(* Logix 5000 AddOnInstructionDefinition export EipIoDataMapping_PAL_EIP; software revision 37.00 *)

TYPE PneumaticAutomationLink_UDT :
STRUCT
   sts_DiagnosticData : SINT;
   sts_DigitalInput_8pt_Module : SINT[16];
   sts_AnalogInput : INT[16];   // Raw Data
   sts_DigitalInput_16pt_Module : INT[8];
   sts_TemperatureInput : INT[16];   // Implied Decimal
   cmd_Valves : BOOL[128];   // Solenoids
   cmd_DigitalOutput_8pt_Module : SINT[16];
   cmd_DigitalOutput_6pt_Module : SINT[22];   // w/ Auxiliary Power
   cmd_AnalogOutput : INT[16];   // Raw Data
   cmd_DigitalOutput_16pt_Module : INT[8];
END_STRUCT
END_TYPE

ADD_ON_INSTRUCTION EipIoDataMapping_PAL_EIP   (* revision 1.0, vendor Automationdirect.com *)
// This Add-On Instruction unpacks raw Input Data (T->O) from an array and maps this data into meaningful device related status tags for the user. Likewise, the AOI also maps meaningful device related command tags and packs the data into the raw Output Data (O->T) array.
// The purpose of the Add-On Instruction is to simplify the mapping (packing/unpacking) of the raw Input/Output Data. For operation of the drive, the user must provide their own logic.
// Revision note:
// Created in v37.00.00
// Version: 1.0
// - Initial version of the new Add-On Instruction format.
// 2025/06/20
VAR_IN_OUT
   mod_EipInputData : _054B:PAL_EIP_D8303EE7:I:0; {required}   // Module defined using SINT data type
   mod_EipOutputData : _054B:PAL_EIP_3E1CE89C:O:0; {required}   // Module defined using SINT data type
   ref_InstanceOfPal : PneumaticAutomationLink_UDT; {required}   // Reference to an instance of the PneumaticAutomationLink_UDT
END_VAR

ROUTINE Logic   (* ladder *)
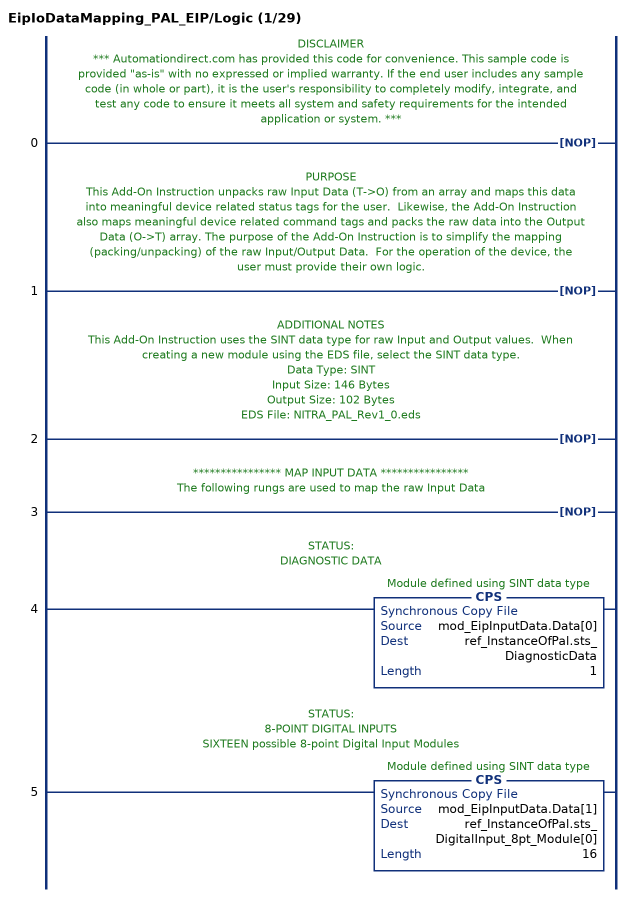
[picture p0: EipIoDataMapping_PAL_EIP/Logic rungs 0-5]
   // DISCLAIMER
   // *** Automationdirect.com has provided this code for convenience. This sample code is provided "as-is" with no expressed or implied warranty. If the end user includes any sample code (in whole or part), it is the user's responsibility to completely modify, integrate, and test any code to ensure it meets all system and safety requirements for the intended application or system. ***
   0: NOP();
   // PURPOSE
   // This Add-On Instruction unpacks raw Input Data (T->O) from an array and maps this data into meaningful device related status tags for the user.  Likewise, the Add-On Instruction also maps meaningful device related command tags and packs the raw data into the Output Data (O->T) array. The purpose of the Add-On Instruction is to simplify the mapping (packing/unpacking) of the raw Input/Output Data.  For the operation of the device, the user must provide their own logic.
   1: NOP();
   // ADDITIONAL NOTES
   // This Add-On Instruction uses the SINT data type for raw Input and Output values.  When creating a new module using the EDS file, select the SINT data type.
   // Data Type: SINT
   // Input Size: 146 Bytes
   // Output Size: 102 Bytes
   // EDS File: NITRA_PAL_Rev1_0.eds
   2: NOP();
   // **************** MAP INPUT DATA ****************
   // The following rungs are used to map the raw Input Data
   3: NOP();
   // STATUS:
   // DIAGNOSTIC DATA
   4: CPS(mod_EipInputData.Data[0],ref_InstanceOfPal.sts_DiagnosticData,1);
   // STATUS:
   // 8-POINT DIGITAL INPUTS
   // SIXTEEN possible 8-point Digital Input Modules
   5: CPS(mod_EipInputData.Data[1],ref_InstanceOfPal.sts_DigitalInput_8pt_Module[0],16);
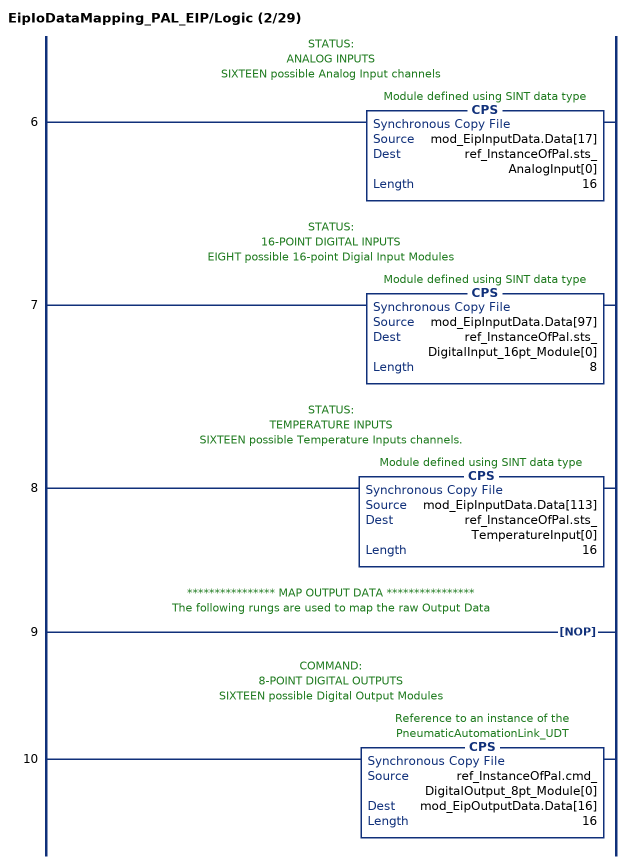
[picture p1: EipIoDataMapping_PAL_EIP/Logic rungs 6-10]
   // STATUS:
   // ANALOG INPUTS
   // SIXTEEN possible Analog Input channels
   6: CPS(mod_EipInputData.Data[17],ref_InstanceOfPal.sts_AnalogInput[0],16);
   // STATUS:
   // 16-POINT DIGITAL INPUTS
   // EIGHT possible 16-point Digial Input Modules
   7: CPS(mod_EipInputData.Data[97],ref_InstanceOfPal.sts_DigitalInput_16pt_Module[0],8);
   // STATUS:
   // TEMPERATURE INPUTS
   // SIXTEEN possible Temperature Inputs channels.
   8: CPS(mod_EipInputData.Data[113],ref_InstanceOfPal.sts_TemperatureInput[0],16);
   // **************** MAP OUTPUT DATA ****************
   // The following rungs are used to map the raw Output Data
   9: NOP();
   // COMMAND:
   // 8-POINT DIGITAL OUTPUTS
   // SIXTEEN possible Digital Output Modules
   10: CPS(ref_InstanceOfPal.cmd_DigitalOutput_8pt_Module[0],mod_EipOutputData.Data[16],16);
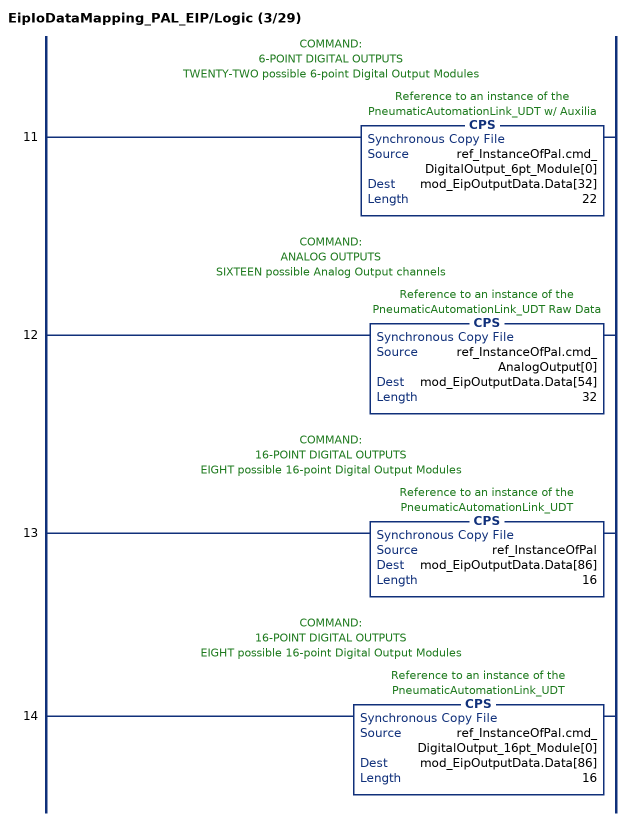
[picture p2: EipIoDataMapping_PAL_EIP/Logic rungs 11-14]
   // COMMAND:
   // 6-POINT DIGITAL OUTPUTS
   // TWENTY-TWO possible 6-point Digital Output Modules
   11: CPS(ref_InstanceOfPal.cmd_DigitalOutput_6pt_Module[0],mod_EipOutputData.Data[32],22);
   // COMMAND:
   // ANALOG OUTPUTS
   // SIXTEEN possible Analog Output channels
   12: CPS(ref_InstanceOfPal.cmd_AnalogOutput[0],mod_EipOutputData.Data[54],32);
   // COMMAND:
   // 16-POINT DIGITAL OUTPUTS
   // EIGHT possible 16-point Digital Output Modules
   13: CPS(ref_InstanceOfPal,mod_EipOutputData.Data[86],16);
   // COMMAND:
   // 16-POINT DIGITAL OUTPUTS
   // EIGHT possible 16-point Digital Output Modules
   14: CPS(ref_InstanceOfPal.cmd_DigitalOutput_16pt_Module[0],mod_EipOutputData.Data[86],16);
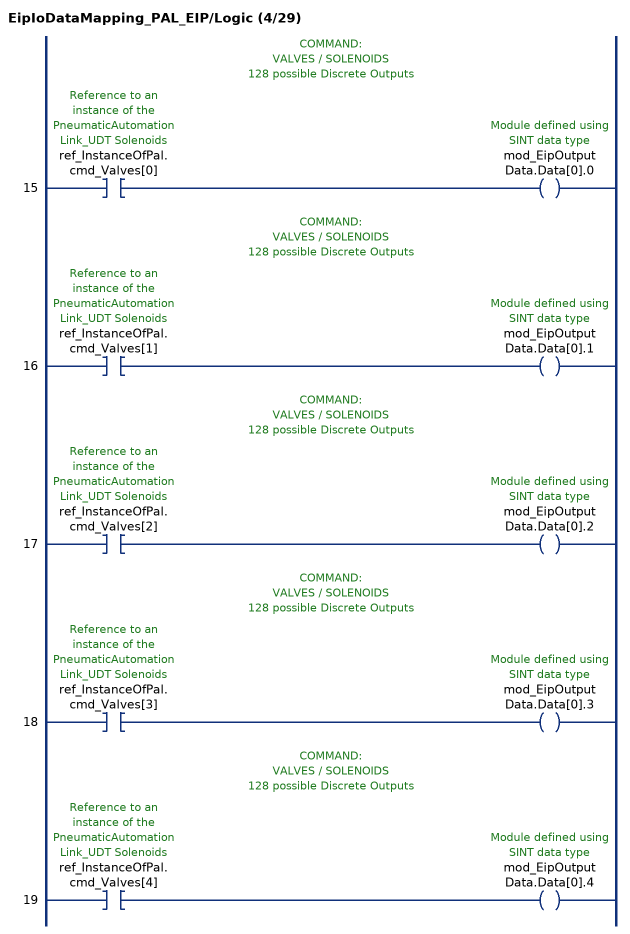
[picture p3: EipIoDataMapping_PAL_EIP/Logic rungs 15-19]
   // COMMAND:
   // VALVES / SOLENOIDS
   // 128 possible Discrete Outputs
   15: XIC(ref_InstanceOfPal.cmd_Valves[0])OTE(mod_EipOutputData.Data[0].0);
   // COMMAND:
   // VALVES / SOLENOIDS
   // 128 possible Discrete Outputs
   16: XIC(ref_InstanceOfPal.cmd_Valves[1])OTE(mod_EipOutputData.Data[0].1);
   // COMMAND:
   // VALVES / SOLENOIDS
   // 128 possible Discrete Outputs
   17: XIC(ref_InstanceOfPal.cmd_Valves[2])OTE(mod_EipOutputData.Data[0].2);
   // COMMAND:
   // VALVES / SOLENOIDS
   // 128 possible Discrete Outputs
   18: XIC(ref_InstanceOfPal.cmd_Valves[3])OTE(mod_EipOutputData.Data[0].3);
   // COMMAND:
   // VALVES / SOLENOIDS
   // 128 possible Discrete Outputs
   19: XIC(ref_InstanceOfPal.cmd_Valves[4])OTE(mod_EipOutputData.Data[0].4);
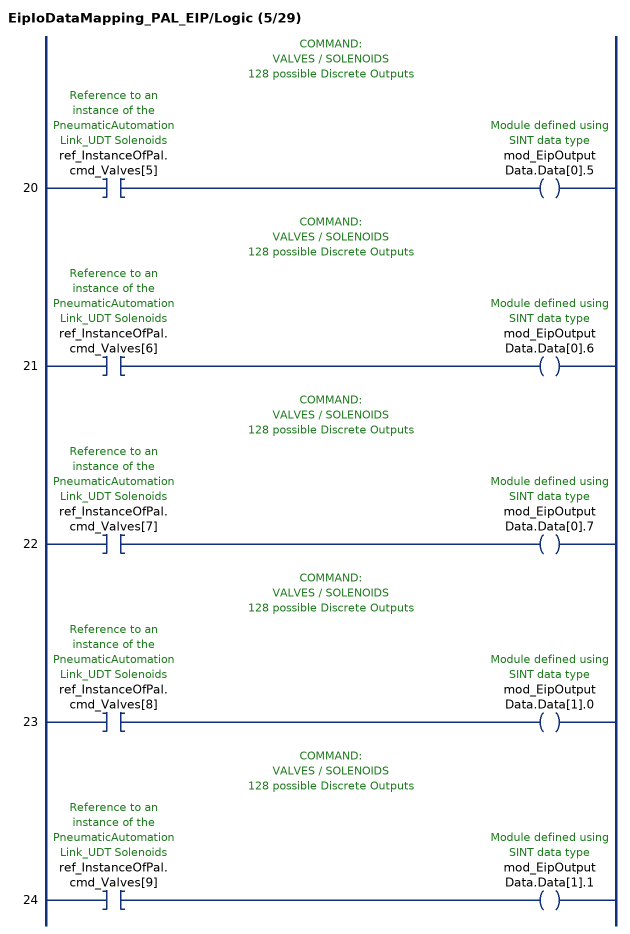
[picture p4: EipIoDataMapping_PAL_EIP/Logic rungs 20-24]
   // COMMAND:
   // VALVES / SOLENOIDS
   // 128 possible Discrete Outputs
   20: XIC(ref_InstanceOfPal.cmd_Valves[5])OTE(mod_EipOutputData.Data[0].5);
   // COMMAND:
   // VALVES / SOLENOIDS
   // 128 possible Discrete Outputs
   21: XIC(ref_InstanceOfPal.cmd_Valves[6])OTE(mod_EipOutputData.Data[0].6);
   // COMMAND:
   // VALVES / SOLENOIDS
   // 128 possible Discrete Outputs
   22: XIC(ref_InstanceOfPal.cmd_Valves[7])OTE(mod_EipOutputData.Data[0].7);
   // COMMAND:
   // VALVES / SOLENOIDS
   // 128 possible Discrete Outputs
   23: XIC(ref_InstanceOfPal.cmd_Valves[8])OTE(mod_EipOutputData.Data[1].0);
   // COMMAND:
   // VALVES / SOLENOIDS
   // 128 possible Discrete Outputs
   24: XIC(ref_InstanceOfPal.cmd_Valves[9])OTE(mod_EipOutputData.Data[1].1);
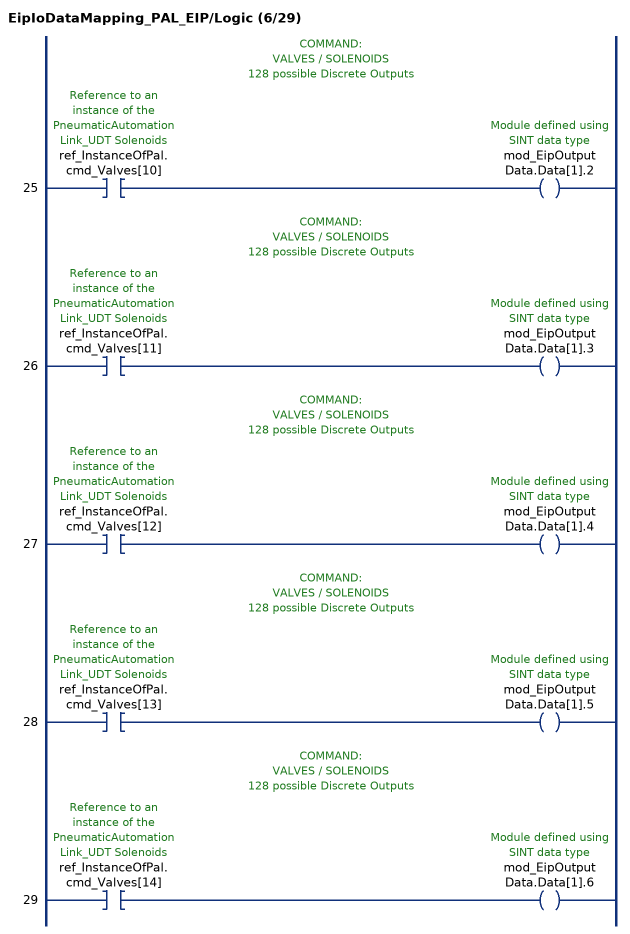
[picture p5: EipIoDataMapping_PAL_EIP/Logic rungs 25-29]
   // COMMAND:
   // VALVES / SOLENOIDS
   // 128 possible Discrete Outputs
   25: XIC(ref_InstanceOfPal.cmd_Valves[10])OTE(mod_EipOutputData.Data[1].2);
   // COMMAND:
   // VALVES / SOLENOIDS
   // 128 possible Discrete Outputs
   26: XIC(ref_InstanceOfPal.cmd_Valves[11])OTE(mod_EipOutputData.Data[1].3);
   // COMMAND:
   // VALVES / SOLENOIDS
   // 128 possible Discrete Outputs
   27: XIC(ref_InstanceOfPal.cmd_Valves[12])OTE(mod_EipOutputData.Data[1].4);
   // COMMAND:
   // VALVES / SOLENOIDS
   // 128 possible Discrete Outputs
   28: XIC(ref_InstanceOfPal.cmd_Valves[13])OTE(mod_EipOutputData.Data[1].5);
   // COMMAND:
   // VALVES / SOLENOIDS
   // 128 possible Discrete Outputs
   29: XIC(ref_InstanceOfPal.cmd_Valves[14])OTE(mod_EipOutputData.Data[1].6);
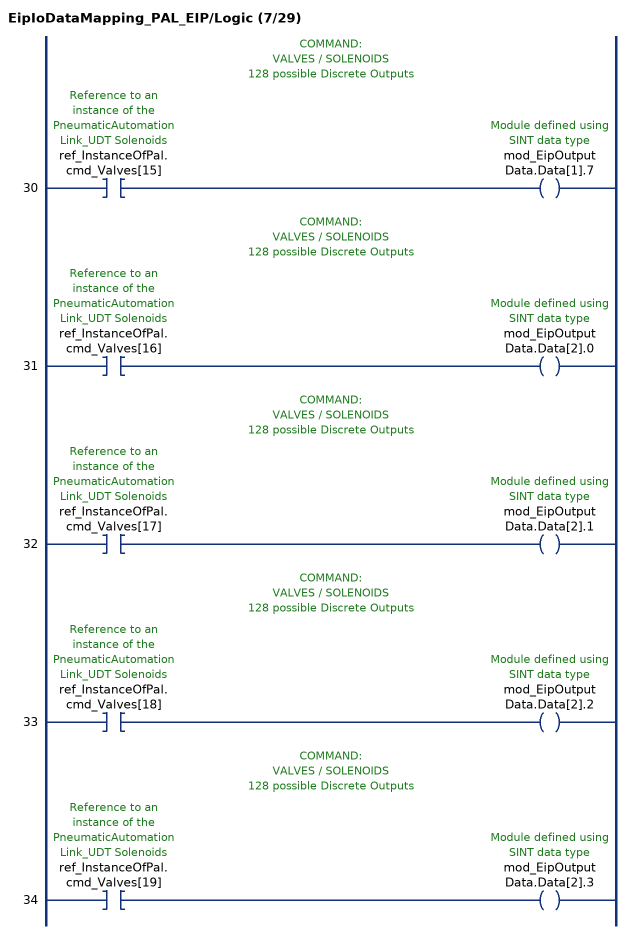
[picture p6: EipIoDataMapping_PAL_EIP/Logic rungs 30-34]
   // COMMAND:
   // VALVES / SOLENOIDS
   // 128 possible Discrete Outputs
   30: XIC(ref_InstanceOfPal.cmd_Valves[15])OTE(mod_EipOutputData.Data[1].7);
   // COMMAND:
   // VALVES / SOLENOIDS
   // 128 possible Discrete Outputs
   31: XIC(ref_InstanceOfPal.cmd_Valves[16])OTE(mod_EipOutputData.Data[2].0);
   // COMMAND:
   // VALVES / SOLENOIDS
   // 128 possible Discrete Outputs
   32: XIC(ref_InstanceOfPal.cmd_Valves[17])OTE(mod_EipOutputData.Data[2].1);
   // COMMAND:
   // VALVES / SOLENOIDS
   // 128 possible Discrete Outputs
   33: XIC(ref_InstanceOfPal.cmd_Valves[18])OTE(mod_EipOutputData.Data[2].2);
   // COMMAND:
   // VALVES / SOLENOIDS
   // 128 possible Discrete Outputs
   34: XIC(ref_InstanceOfPal.cmd_Valves[19])OTE(mod_EipOutputData.Data[2].3);
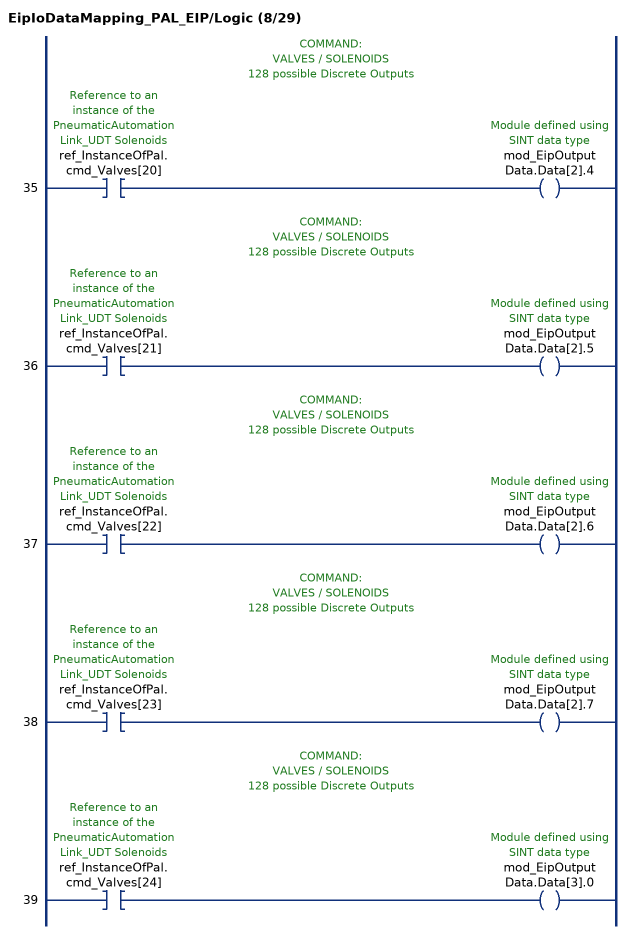
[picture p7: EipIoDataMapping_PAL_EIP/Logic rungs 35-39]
   // COMMAND:
   // VALVES / SOLENOIDS
   // 128 possible Discrete Outputs
   35: XIC(ref_InstanceOfPal.cmd_Valves[20])OTE(mod_EipOutputData.Data[2].4);
   // COMMAND:
   // VALVES / SOLENOIDS
   // 128 possible Discrete Outputs
   36: XIC(ref_InstanceOfPal.cmd_Valves[21])OTE(mod_EipOutputData.Data[2].5);
   // COMMAND:
   // VALVES / SOLENOIDS
   // 128 possible Discrete Outputs
   37: XIC(ref_InstanceOfPal.cmd_Valves[22])OTE(mod_EipOutputData.Data[2].6);
   // COMMAND:
   // VALVES / SOLENOIDS
   // 128 possible Discrete Outputs
   38: XIC(ref_InstanceOfPal.cmd_Valves[23])OTE(mod_EipOutputData.Data[2].7);
   // COMMAND:
   // VALVES / SOLENOIDS
   // 128 possible Discrete Outputs
   39: XIC(ref_InstanceOfPal.cmd_Valves[24])OTE(mod_EipOutputData.Data[3].0);
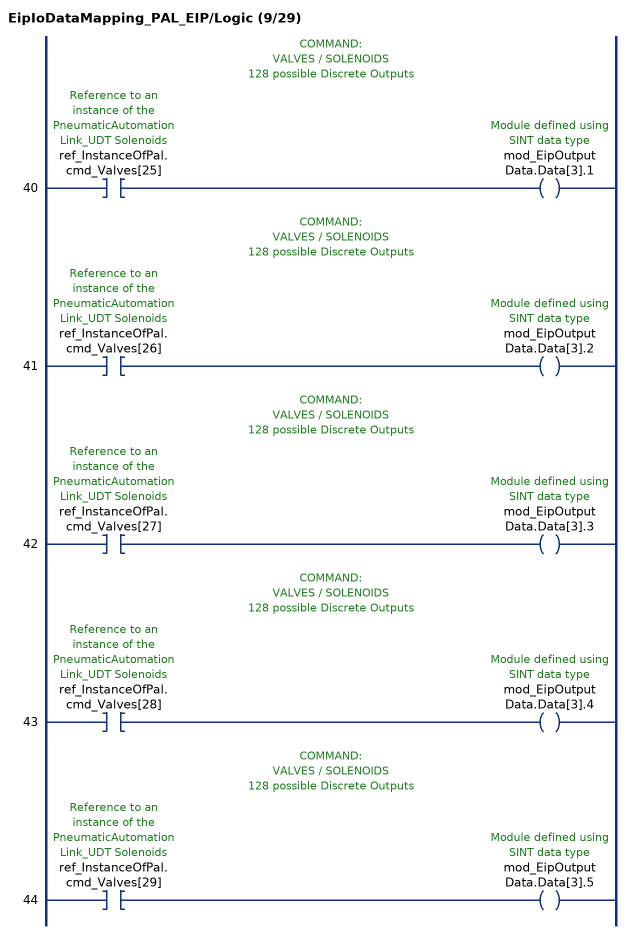
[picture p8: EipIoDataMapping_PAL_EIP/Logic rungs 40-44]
   // COMMAND:
   // VALVES / SOLENOIDS
   // 128 possible Discrete Outputs
   40: XIC(ref_InstanceOfPal.cmd_Valves[25])OTE(mod_EipOutputData.Data[3].1);
   // COMMAND:
   // VALVES / SOLENOIDS
   // 128 possible Discrete Outputs
   41: XIC(ref_InstanceOfPal.cmd_Valves[26])OTE(mod_EipOutputData.Data[3].2);
   // COMMAND:
   // VALVES / SOLENOIDS
   // 128 possible Discrete Outputs
   42: XIC(ref_InstanceOfPal.cmd_Valves[27])OTE(mod_EipOutputData.Data[3].3);
   // COMMAND:
   // VALVES / SOLENOIDS
   // 128 possible Discrete Outputs
   43: XIC(ref_InstanceOfPal.cmd_Valves[28])OTE(mod_EipOutputData.Data[3].4);
   // COMMAND:
   // VALVES / SOLENOIDS
   // 128 possible Discrete Outputs
   44: XIC(ref_InstanceOfPal.cmd_Valves[29])OTE(mod_EipOutputData.Data[3].5);
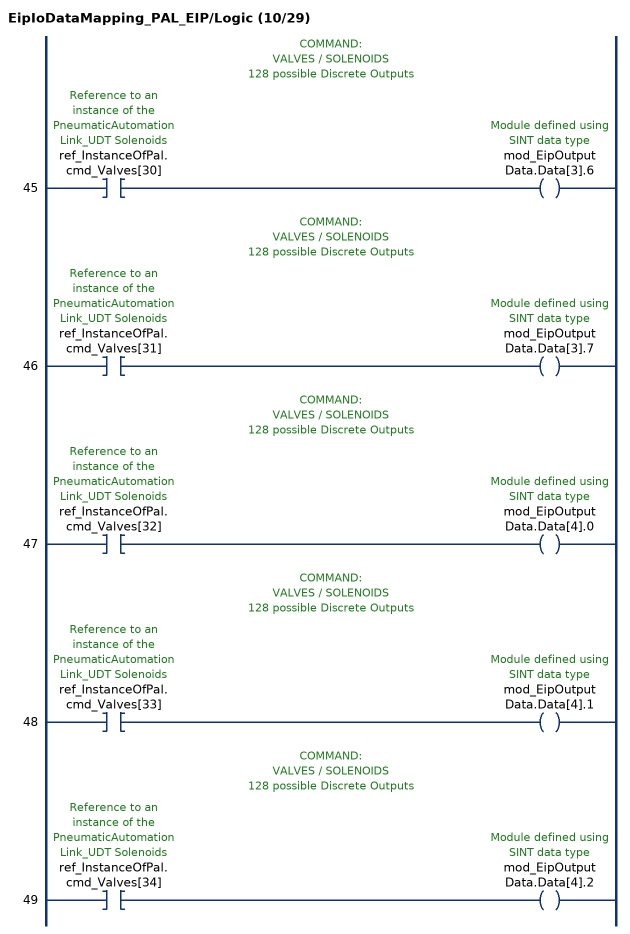
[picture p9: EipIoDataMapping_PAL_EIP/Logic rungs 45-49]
   // COMMAND:
   // VALVES / SOLENOIDS
   // 128 possible Discrete Outputs
   45: XIC(ref_InstanceOfPal.cmd_Valves[30])OTE(mod_EipOutputData.Data[3].6);
   // COMMAND:
   // VALVES / SOLENOIDS
   // 128 possible Discrete Outputs
   46: XIC(ref_InstanceOfPal.cmd_Valves[31])OTE(mod_EipOutputData.Data[3].7);
   // COMMAND:
   // VALVES / SOLENOIDS
   // 128 possible Discrete Outputs
   47: XIC(ref_InstanceOfPal.cmd_Valves[32])OTE(mod_EipOutputData.Data[4].0);
   // COMMAND:
   // VALVES / SOLENOIDS
   // 128 possible Discrete Outputs
   48: XIC(ref_InstanceOfPal.cmd_Valves[33])OTE(mod_EipOutputData.Data[4].1);
   // COMMAND:
   // VALVES / SOLENOIDS
   // 128 possible Discrete Outputs
   49: XIC(ref_InstanceOfPal.cmd_Valves[34])OTE(mod_EipOutputData.Data[4].2);
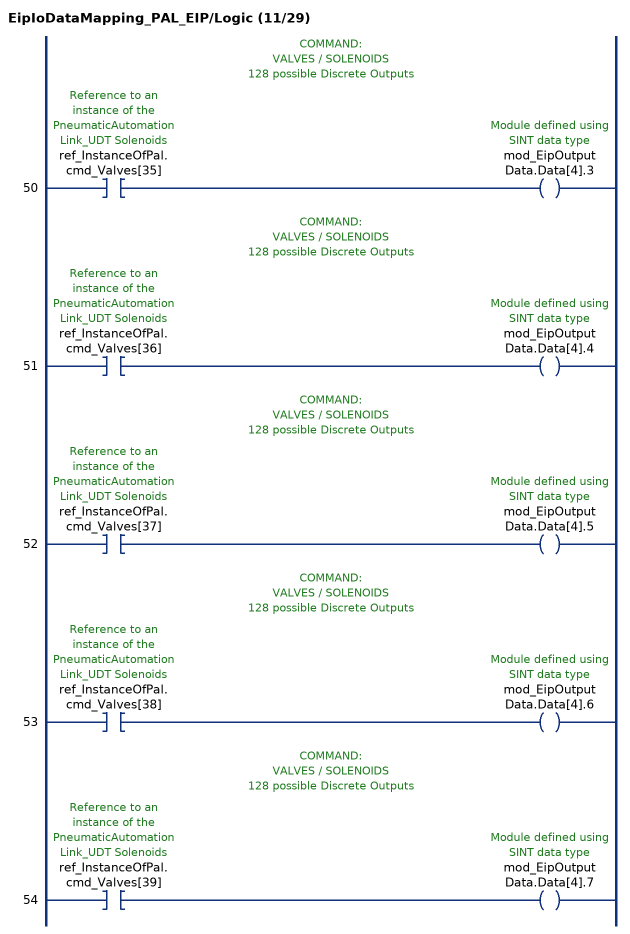
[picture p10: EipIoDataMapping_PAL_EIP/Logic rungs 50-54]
   // COMMAND:
   // VALVES / SOLENOIDS
   // 128 possible Discrete Outputs
   50: XIC(ref_InstanceOfPal.cmd_Valves[35])OTE(mod_EipOutputData.Data[4].3);
   // COMMAND:
   // VALVES / SOLENOIDS
   // 128 possible Discrete Outputs
   51: XIC(ref_InstanceOfPal.cmd_Valves[36])OTE(mod_EipOutputData.Data[4].4);
   // COMMAND:
   // VALVES / SOLENOIDS
   // 128 possible Discrete Outputs
   52: XIC(ref_InstanceOfPal.cmd_Valves[37])OTE(mod_EipOutputData.Data[4].5);
   // COMMAND:
   // VALVES / SOLENOIDS
   // 128 possible Discrete Outputs
   53: XIC(ref_InstanceOfPal.cmd_Valves[38])OTE(mod_EipOutputData.Data[4].6);
   // COMMAND:
   // VALVES / SOLENOIDS
   // 128 possible Discrete Outputs
   54: XIC(ref_InstanceOfPal.cmd_Valves[39])OTE(mod_EipOutputData.Data[4].7);
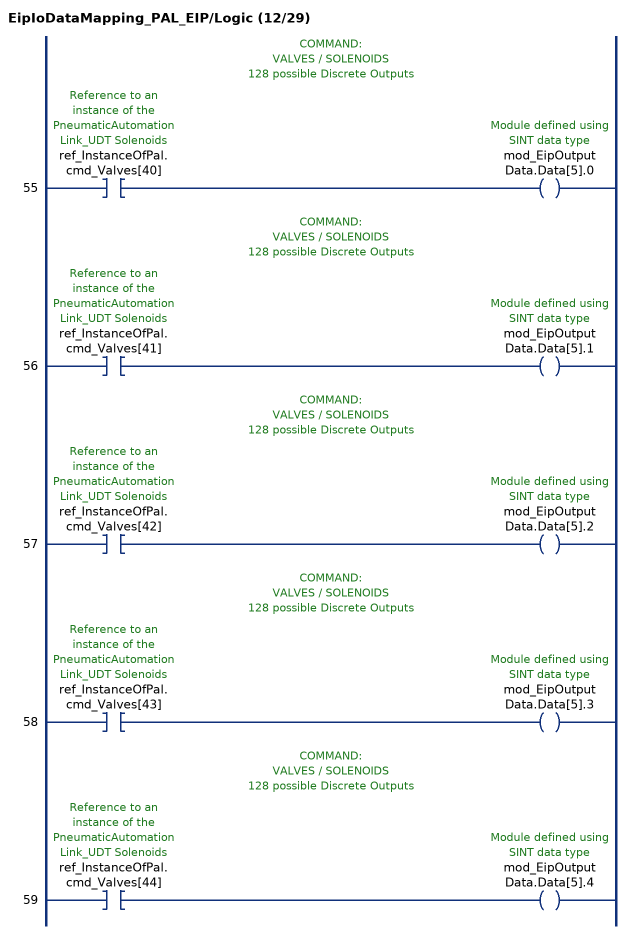
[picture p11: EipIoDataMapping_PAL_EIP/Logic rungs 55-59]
   // COMMAND:
   // VALVES / SOLENOIDS
   // 128 possible Discrete Outputs
   55: XIC(ref_InstanceOfPal.cmd_Valves[40])OTE(mod_EipOutputData.Data[5].0);
   // COMMAND:
   // VALVES / SOLENOIDS
   // 128 possible Discrete Outputs
   56: XIC(ref_InstanceOfPal.cmd_Valves[41])OTE(mod_EipOutputData.Data[5].1);
   // COMMAND:
   // VALVES / SOLENOIDS
   // 128 possible Discrete Outputs
   57: XIC(ref_InstanceOfPal.cmd_Valves[42])OTE(mod_EipOutputData.Data[5].2);
   // COMMAND:
   // VALVES / SOLENOIDS
   // 128 possible Discrete Outputs
   58: XIC(ref_InstanceOfPal.cmd_Valves[43])OTE(mod_EipOutputData.Data[5].3);
   // COMMAND:
   // VALVES / SOLENOIDS
   // 128 possible Discrete Outputs
   59: XIC(ref_InstanceOfPal.cmd_Valves[44])OTE(mod_EipOutputData.Data[5].4);
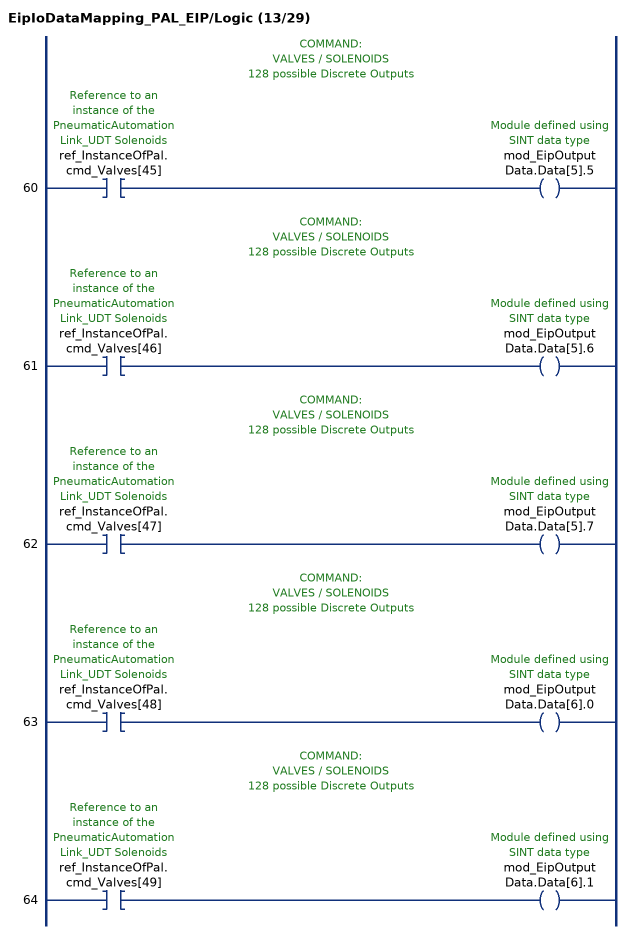
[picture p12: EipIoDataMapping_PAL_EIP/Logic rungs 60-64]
   // COMMAND:
   // VALVES / SOLENOIDS
   // 128 possible Discrete Outputs
   60: XIC(ref_InstanceOfPal.cmd_Valves[45])OTE(mod_EipOutputData.Data[5].5);
   // COMMAND:
   // VALVES / SOLENOIDS
   // 128 possible Discrete Outputs
   61: XIC(ref_InstanceOfPal.cmd_Valves[46])OTE(mod_EipOutputData.Data[5].6);
   // COMMAND:
   // VALVES / SOLENOIDS
   // 128 possible Discrete Outputs
   62: XIC(ref_InstanceOfPal.cmd_Valves[47])OTE(mod_EipOutputData.Data[5].7);
   // COMMAND:
   // VALVES / SOLENOIDS
   // 128 possible Discrete Outputs
   63: XIC(ref_InstanceOfPal.cmd_Valves[48])OTE(mod_EipOutputData.Data[6].0);
   // COMMAND:
   // VALVES / SOLENOIDS
   // 128 possible Discrete Outputs
   64: XIC(ref_InstanceOfPal.cmd_Valves[49])OTE(mod_EipOutputData.Data[6].1);
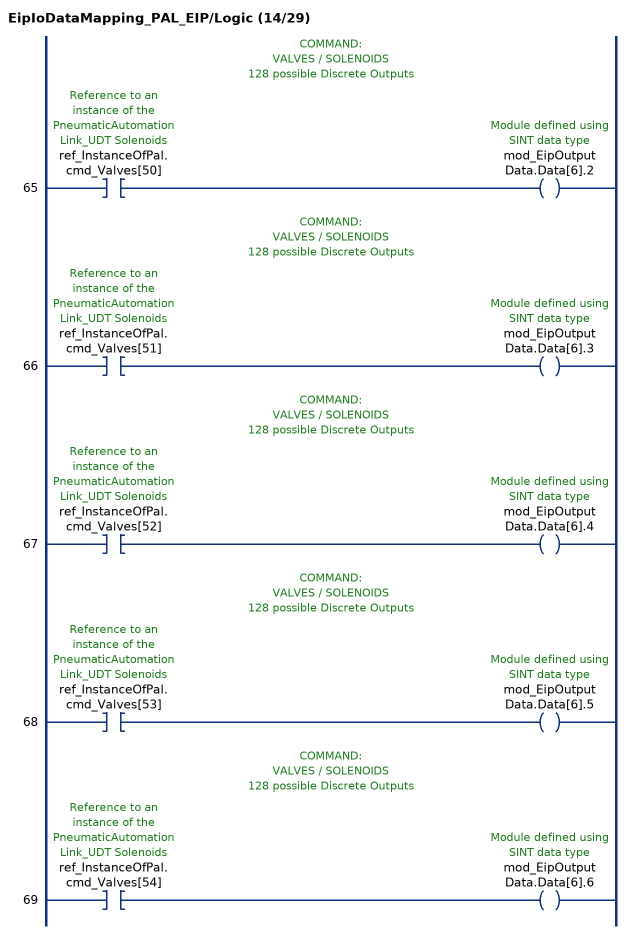
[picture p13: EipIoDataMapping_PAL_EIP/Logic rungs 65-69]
   // COMMAND:
   // VALVES / SOLENOIDS
   // 128 possible Discrete Outputs
   65: XIC(ref_InstanceOfPal.cmd_Valves[50])OTE(mod_EipOutputData.Data[6].2);
   // COMMAND:
   // VALVES / SOLENOIDS
   // 128 possible Discrete Outputs
   66: XIC(ref_InstanceOfPal.cmd_Valves[51])OTE(mod_EipOutputData.Data[6].3);
   // COMMAND:
   // VALVES / SOLENOIDS
   // 128 possible Discrete Outputs
   67: XIC(ref_InstanceOfPal.cmd_Valves[52])OTE(mod_EipOutputData.Data[6].4);
   // COMMAND:
   // VALVES / SOLENOIDS
   // 128 possible Discrete Outputs
   68: XIC(ref_InstanceOfPal.cmd_Valves[53])OTE(mod_EipOutputData.Data[6].5);
   // COMMAND:
   // VALVES / SOLENOIDS
   // 128 possible Discrete Outputs
   69: XIC(ref_InstanceOfPal.cmd_Valves[54])OTE(mod_EipOutputData.Data[6].6);
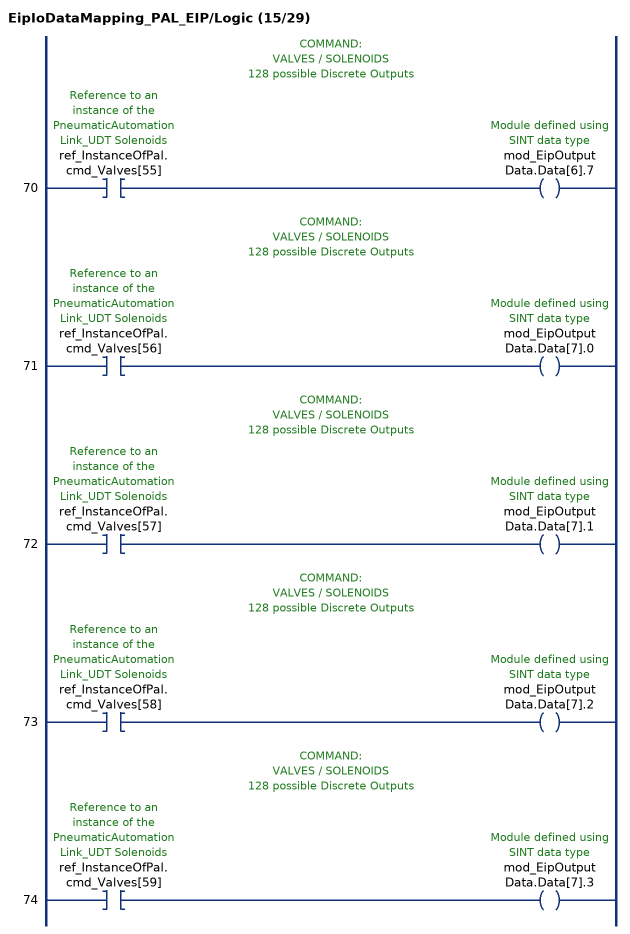
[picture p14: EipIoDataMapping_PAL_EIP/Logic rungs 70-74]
   // COMMAND:
   // VALVES / SOLENOIDS
   // 128 possible Discrete Outputs
   70: XIC(ref_InstanceOfPal.cmd_Valves[55])OTE(mod_EipOutputData.Data[6].7);
   // COMMAND:
   // VALVES / SOLENOIDS
   // 128 possible Discrete Outputs
   71: XIC(ref_InstanceOfPal.cmd_Valves[56])OTE(mod_EipOutputData.Data[7].0);
   // COMMAND:
   // VALVES / SOLENOIDS
   // 128 possible Discrete Outputs
   72: XIC(ref_InstanceOfPal.cmd_Valves[57])OTE(mod_EipOutputData.Data[7].1);
   // COMMAND:
   // VALVES / SOLENOIDS
   // 128 possible Discrete Outputs
   73: XIC(ref_InstanceOfPal.cmd_Valves[58])OTE(mod_EipOutputData.Data[7].2);
   // COMMAND:
   // VALVES / SOLENOIDS
   // 128 possible Discrete Outputs
   74: XIC(ref_InstanceOfPal.cmd_Valves[59])OTE(mod_EipOutputData.Data[7].3);
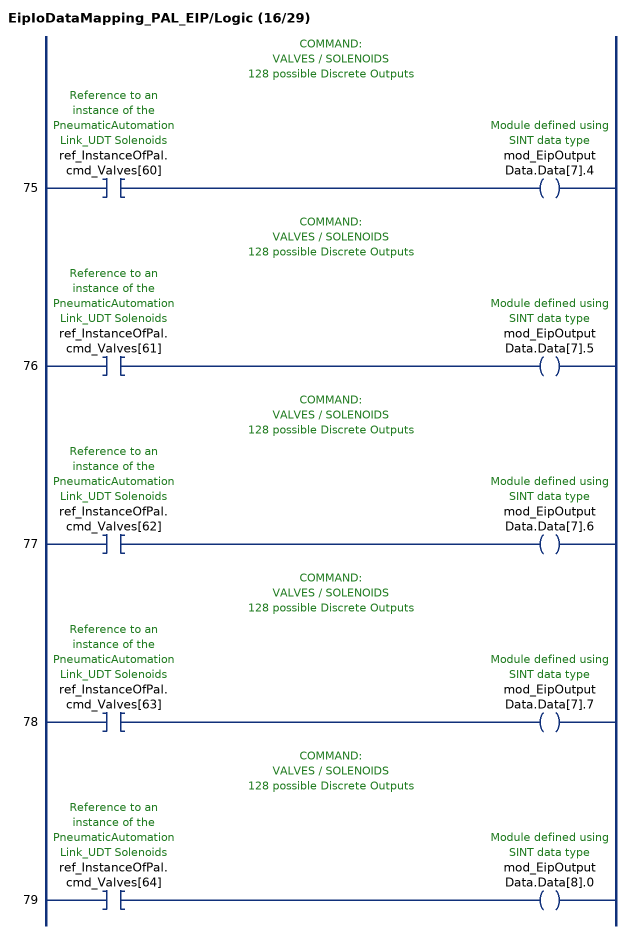
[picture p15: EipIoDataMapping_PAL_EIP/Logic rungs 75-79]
   // COMMAND:
   // VALVES / SOLENOIDS
   // 128 possible Discrete Outputs
   75: XIC(ref_InstanceOfPal.cmd_Valves[60])OTE(mod_EipOutputData.Data[7].4);
   // COMMAND:
   // VALVES / SOLENOIDS
   // 128 possible Discrete Outputs
   76: XIC(ref_InstanceOfPal.cmd_Valves[61])OTE(mod_EipOutputData.Data[7].5);
   // COMMAND:
   // VALVES / SOLENOIDS
   // 128 possible Discrete Outputs
   77: XIC(ref_InstanceOfPal.cmd_Valves[62])OTE(mod_EipOutputData.Data[7].6);
   // COMMAND:
   // VALVES / SOLENOIDS
   // 128 possible Discrete Outputs
   78: XIC(ref_InstanceOfPal.cmd_Valves[63])OTE(mod_EipOutputData.Data[7].7);
   // COMMAND:
   // VALVES / SOLENOIDS
   // 128 possible Discrete Outputs
   79: XIC(ref_InstanceOfPal.cmd_Valves[64])OTE(mod_EipOutputData.Data[8].0);
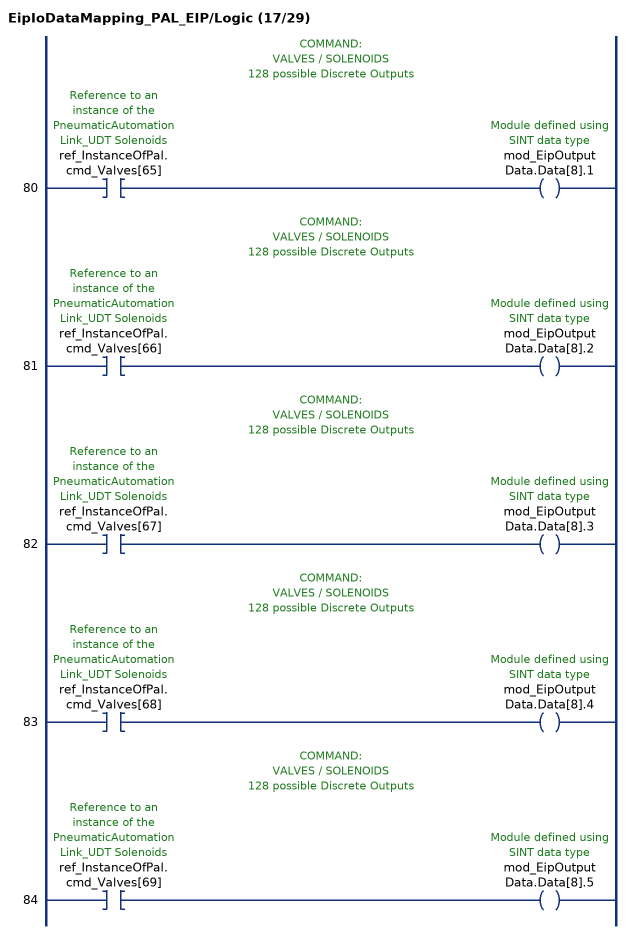
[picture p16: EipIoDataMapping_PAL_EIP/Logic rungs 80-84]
   // COMMAND:
   // VALVES / SOLENOIDS
   // 128 possible Discrete Outputs
   80: XIC(ref_InstanceOfPal.cmd_Valves[65])OTE(mod_EipOutputData.Data[8].1);
   // COMMAND:
   // VALVES / SOLENOIDS
   // 128 possible Discrete Outputs
   81: XIC(ref_InstanceOfPal.cmd_Valves[66])OTE(mod_EipOutputData.Data[8].2);
   // COMMAND:
   // VALVES / SOLENOIDS
   // 128 possible Discrete Outputs
   82: XIC(ref_InstanceOfPal.cmd_Valves[67])OTE(mod_EipOutputData.Data[8].3);
   // COMMAND:
   // VALVES / SOLENOIDS
   // 128 possible Discrete Outputs
   83: XIC(ref_InstanceOfPal.cmd_Valves[68])OTE(mod_EipOutputData.Data[8].4);
   // COMMAND:
   // VALVES / SOLENOIDS
   // 128 possible Discrete Outputs
   84: XIC(ref_InstanceOfPal.cmd_Valves[69])OTE(mod_EipOutputData.Data[8].5);
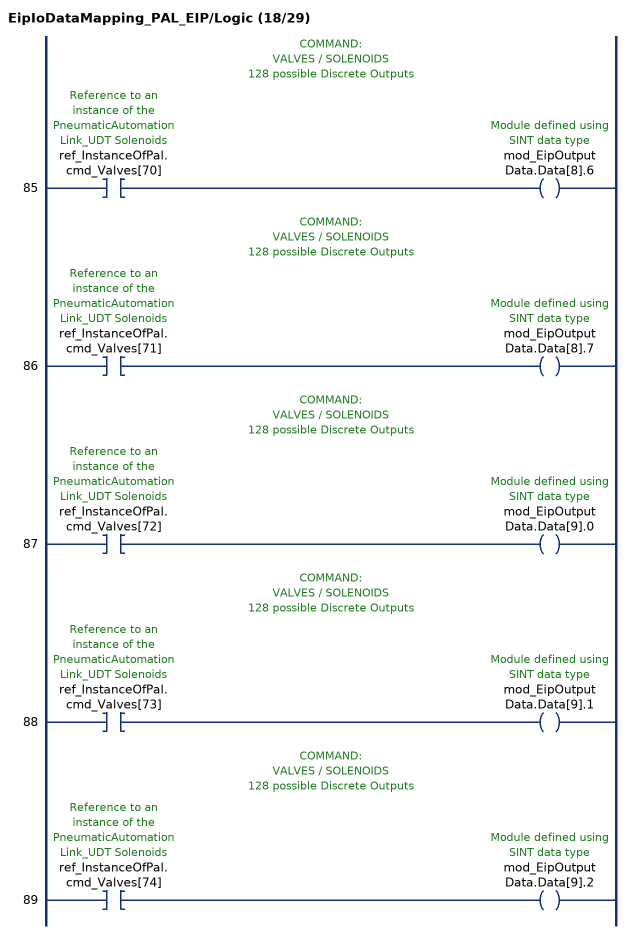
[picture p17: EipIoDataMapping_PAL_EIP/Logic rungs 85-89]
   // COMMAND:
   // VALVES / SOLENOIDS
   // 128 possible Discrete Outputs
   85: XIC(ref_InstanceOfPal.cmd_Valves[70])OTE(mod_EipOutputData.Data[8].6);
   // COMMAND:
   // VALVES / SOLENOIDS
   // 128 possible Discrete Outputs
   86: XIC(ref_InstanceOfPal.cmd_Valves[71])OTE(mod_EipOutputData.Data[8].7);
   // COMMAND:
   // VALVES / SOLENOIDS
   // 128 possible Discrete Outputs
   87: XIC(ref_InstanceOfPal.cmd_Valves[72])OTE(mod_EipOutputData.Data[9].0);
   // COMMAND:
   // VALVES / SOLENOIDS
   // 128 possible Discrete Outputs
   88: XIC(ref_InstanceOfPal.cmd_Valves[73])OTE(mod_EipOutputData.Data[9].1);
   // COMMAND:
   // VALVES / SOLENOIDS
   // 128 possible Discrete Outputs
   89: XIC(ref_InstanceOfPal.cmd_Valves[74])OTE(mod_EipOutputData.Data[9].2);
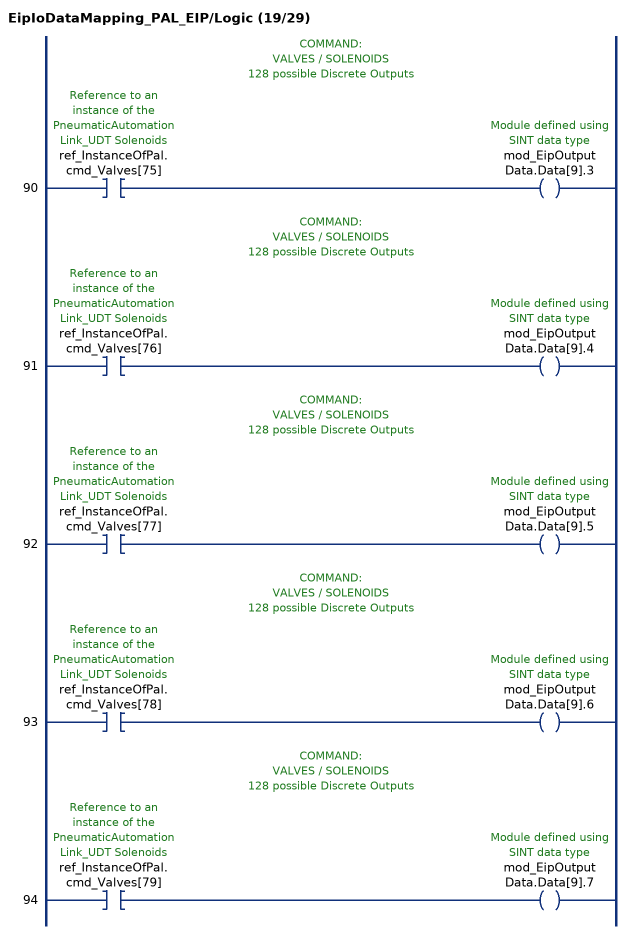
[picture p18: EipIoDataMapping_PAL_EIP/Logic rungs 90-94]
   // COMMAND:
   // VALVES / SOLENOIDS
   // 128 possible Discrete Outputs
   90: XIC(ref_InstanceOfPal.cmd_Valves[75])OTE(mod_EipOutputData.Data[9].3);
   // COMMAND:
   // VALVES / SOLENOIDS
   // 128 possible Discrete Outputs
   91: XIC(ref_InstanceOfPal.cmd_Valves[76])OTE(mod_EipOutputData.Data[9].4);
   // COMMAND:
   // VALVES / SOLENOIDS
   // 128 possible Discrete Outputs
   92: XIC(ref_InstanceOfPal.cmd_Valves[77])OTE(mod_EipOutputData.Data[9].5);
   // COMMAND:
   // VALVES / SOLENOIDS
   // 128 possible Discrete Outputs
   93: XIC(ref_InstanceOfPal.cmd_Valves[78])OTE(mod_EipOutputData.Data[9].6);
   // COMMAND:
   // VALVES / SOLENOIDS
   // 128 possible Discrete Outputs
   94: XIC(ref_InstanceOfPal.cmd_Valves[79])OTE(mod_EipOutputData.Data[9].7);
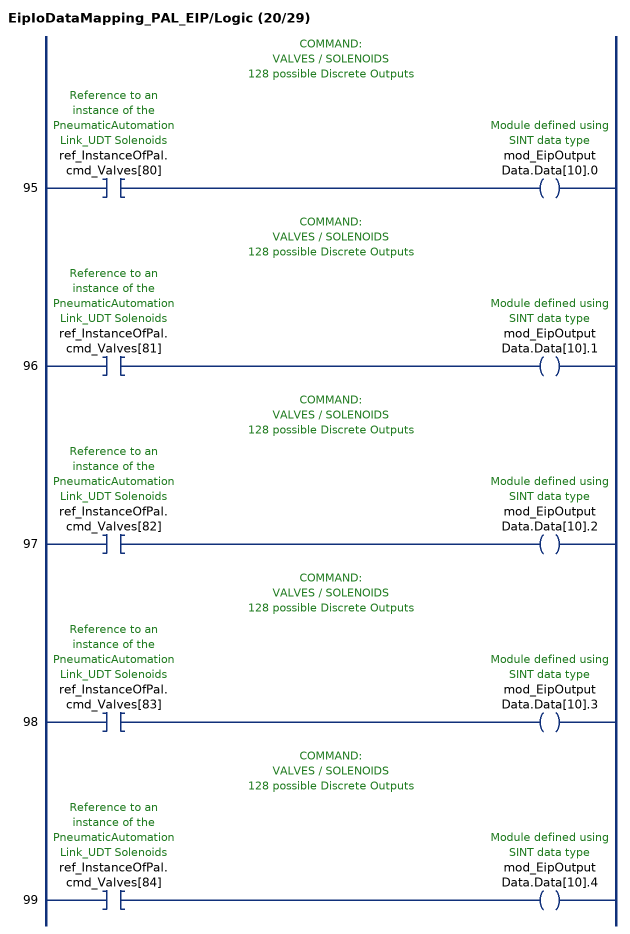
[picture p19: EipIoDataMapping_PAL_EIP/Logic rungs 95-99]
   // COMMAND:
   // VALVES / SOLENOIDS
   // 128 possible Discrete Outputs
   95: XIC(ref_InstanceOfPal.cmd_Valves[80])OTE(mod_EipOutputData.Data[10].0);
   // COMMAND:
   // VALVES / SOLENOIDS
   // 128 possible Discrete Outputs
   96: XIC(ref_InstanceOfPal.cmd_Valves[81])OTE(mod_EipOutputData.Data[10].1);
   // COMMAND:
   // VALVES / SOLENOIDS
   // 128 possible Discrete Outputs
   97: XIC(ref_InstanceOfPal.cmd_Valves[82])OTE(mod_EipOutputData.Data[10].2);
   // COMMAND:
   // VALVES / SOLENOIDS
   // 128 possible Discrete Outputs
   98: XIC(ref_InstanceOfPal.cmd_Valves[83])OTE(mod_EipOutputData.Data[10].3);
   // COMMAND:
   // VALVES / SOLENOIDS
   // 128 possible Discrete Outputs
   99: XIC(ref_InstanceOfPal.cmd_Valves[84])OTE(mod_EipOutputData.Data[10].4);
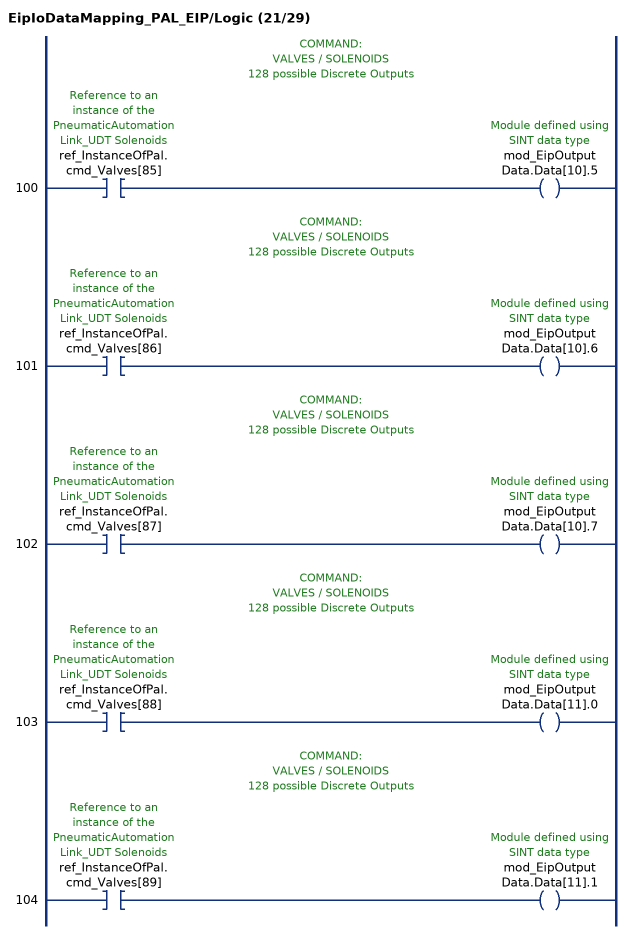
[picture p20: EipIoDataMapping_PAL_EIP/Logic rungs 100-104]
   // COMMAND:
   // VALVES / SOLENOIDS
   // 128 possible Discrete Outputs
   100: XIC(ref_InstanceOfPal.cmd_Valves[85])OTE(mod_EipOutputData.Data[10].5);
   // COMMAND:
   // VALVES / SOLENOIDS
   // 128 possible Discrete Outputs
   101: XIC(ref_InstanceOfPal.cmd_Valves[86])OTE(mod_EipOutputData.Data[10].6);
   // COMMAND:
   // VALVES / SOLENOIDS
   // 128 possible Discrete Outputs
   102: XIC(ref_InstanceOfPal.cmd_Valves[87])OTE(mod_EipOutputData.Data[10].7);
   // COMMAND:
   // VALVES / SOLENOIDS
   // 128 possible Discrete Outputs
   103: XIC(ref_InstanceOfPal.cmd_Valves[88])OTE(mod_EipOutputData.Data[11].0);
   // COMMAND:
   // VALVES / SOLENOIDS
   // 128 possible Discrete Outputs
   104: XIC(ref_InstanceOfPal.cmd_Valves[89])OTE(mod_EipOutputData.Data[11].1);
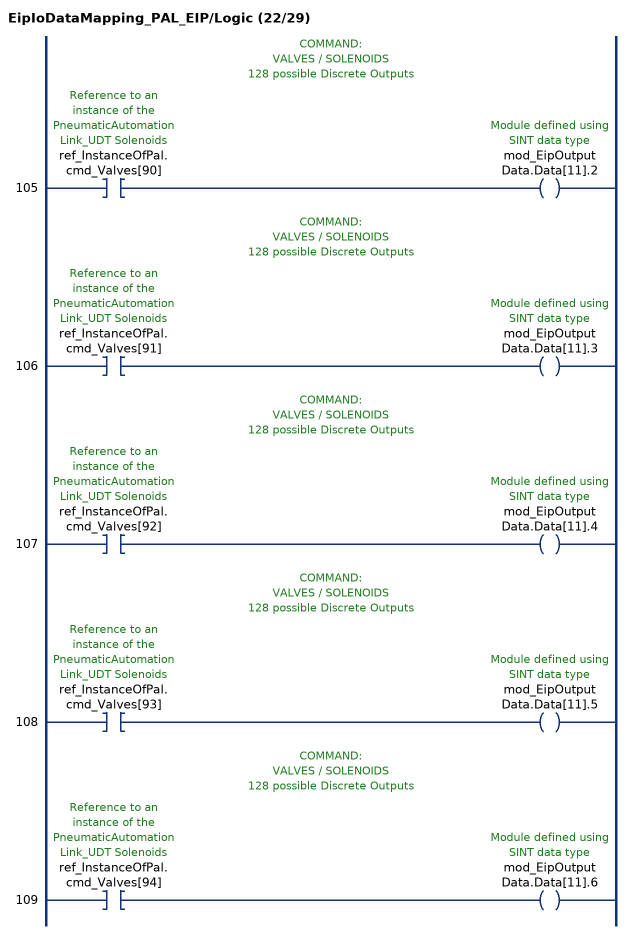
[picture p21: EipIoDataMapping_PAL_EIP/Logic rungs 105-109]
   // COMMAND:
   // VALVES / SOLENOIDS
   // 128 possible Discrete Outputs
   105: XIC(ref_InstanceOfPal.cmd_Valves[90])OTE(mod_EipOutputData.Data[11].2);
   // COMMAND:
   // VALVES / SOLENOIDS
   // 128 possible Discrete Outputs
   106: XIC(ref_InstanceOfPal.cmd_Valves[91])OTE(mod_EipOutputData.Data[11].3);
   // COMMAND:
   // VALVES / SOLENOIDS
   // 128 possible Discrete Outputs
   107: XIC(ref_InstanceOfPal.cmd_Valves[92])OTE(mod_EipOutputData.Data[11].4);
   // COMMAND:
   // VALVES / SOLENOIDS
   // 128 possible Discrete Outputs
   108: XIC(ref_InstanceOfPal.cmd_Valves[93])OTE(mod_EipOutputData.Data[11].5);
   // COMMAND:
   // VALVES / SOLENOIDS
   // 128 possible Discrete Outputs
   109: XIC(ref_InstanceOfPal.cmd_Valves[94])OTE(mod_EipOutputData.Data[11].6);
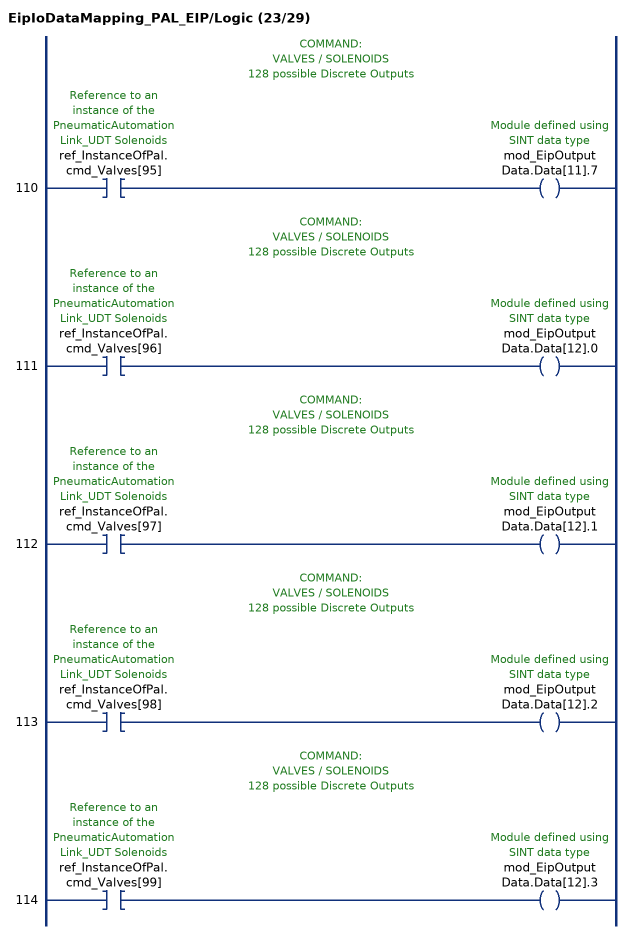
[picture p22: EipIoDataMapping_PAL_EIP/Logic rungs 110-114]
   // COMMAND:
   // VALVES / SOLENOIDS
   // 128 possible Discrete Outputs
   110: XIC(ref_InstanceOfPal.cmd_Valves[95])OTE(mod_EipOutputData.Data[11].7);
   // COMMAND:
   // VALVES / SOLENOIDS
   // 128 possible Discrete Outputs
   111: XIC(ref_InstanceOfPal.cmd_Valves[96])OTE(mod_EipOutputData.Data[12].0);
   // COMMAND:
   // VALVES / SOLENOIDS
   // 128 possible Discrete Outputs
   112: XIC(ref_InstanceOfPal.cmd_Valves[97])OTE(mod_EipOutputData.Data[12].1);
   // COMMAND:
   // VALVES / SOLENOIDS
   // 128 possible Discrete Outputs
   113: XIC(ref_InstanceOfPal.cmd_Valves[98])OTE(mod_EipOutputData.Data[12].2);
   // COMMAND:
   // VALVES / SOLENOIDS
   // 128 possible Discrete Outputs
   114: XIC(ref_InstanceOfPal.cmd_Valves[99])OTE(mod_EipOutputData.Data[12].3);
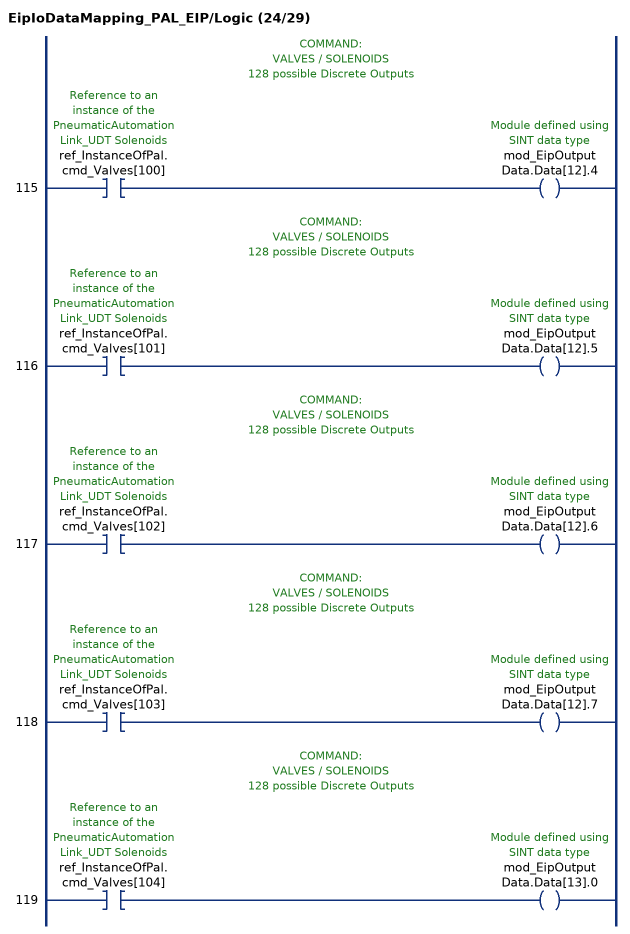
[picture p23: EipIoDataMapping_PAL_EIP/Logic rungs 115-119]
   // COMMAND:
   // VALVES / SOLENOIDS
   // 128 possible Discrete Outputs
   115: XIC(ref_InstanceOfPal.cmd_Valves[100])OTE(mod_EipOutputData.Data[12].4);
   // COMMAND:
   // VALVES / SOLENOIDS
   // 128 possible Discrete Outputs
   116: XIC(ref_InstanceOfPal.cmd_Valves[101])OTE(mod_EipOutputData.Data[12].5);
   // COMMAND:
   // VALVES / SOLENOIDS
   // 128 possible Discrete Outputs
   117: XIC(ref_InstanceOfPal.cmd_Valves[102])OTE(mod_EipOutputData.Data[12].6);
   // COMMAND:
   // VALVES / SOLENOIDS
   // 128 possible Discrete Outputs
   118: XIC(ref_InstanceOfPal.cmd_Valves[103])OTE(mod_EipOutputData.Data[12].7);
   // COMMAND:
   // VALVES / SOLENOIDS
   // 128 possible Discrete Outputs
   119: XIC(ref_InstanceOfPal.cmd_Valves[104])OTE(mod_EipOutputData.Data[13].0);
